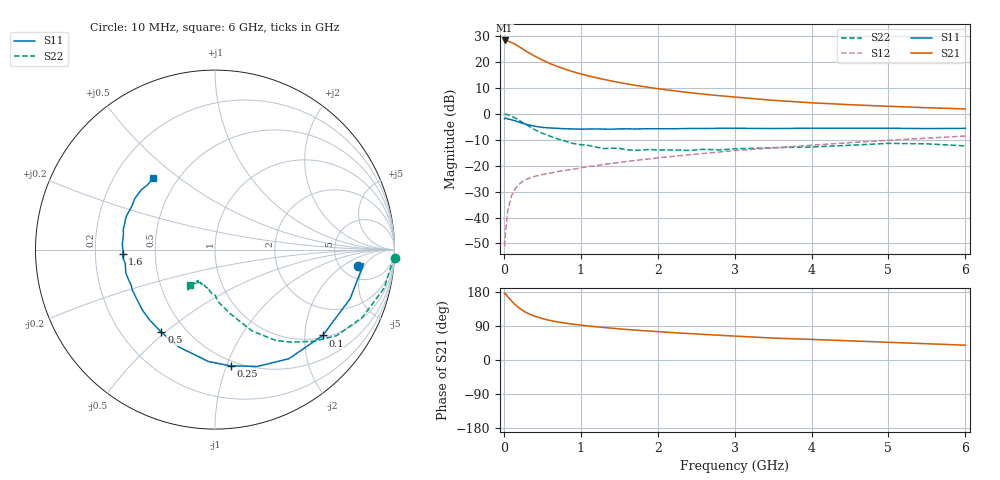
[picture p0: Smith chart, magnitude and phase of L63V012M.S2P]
!  INFINEON TECHNOLOGIES Small Signal Semiconductors
! BFR380L3 , Si-NPN RF-Transistor in TSLP-3-1
!  Vce=3 V,  Ic=12.5 mA
! Common Emitter S-Parameters:  07. March 2005
#  GHz  S  MA  R  50
! f  S11  S21  S12  S22
! GHz  Mag  Ang  Mag  Ang  Mag  Ang  Mag  Ang
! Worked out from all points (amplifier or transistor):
!   36 points, 10 MHz to 6 GHz, reference 50 ohm
!   highest |S21| = 28.4 dB at 10 MHz (marker M1)
!   |S21| within 3 dB of that: start of sweep to 229.8 MHz
!   unconditionally stable (mu >= 1): 2.005 GHz to 4.76 GHz
!   at 250 MHz: K = 0.29, MSG = 25.5 dB, |S12| = -26.0 dB
!   at 1.4 GHz: K = 0.91, MSG = 15.9 dB, |S12| = -19.1 dB
!   at 6 GHz: K = 0.96, MSG = 5.2 dB, |S12| = -8.5 dB
!   S11 on the Smith chart (normalised r, x): 10 MHz: 7.27, -3.66; 100 MHz: 1.06, -2.47; 250 MHz: 0.46, -1.03; 500 MHz: 0.37, -0.49; 1.6 GHz: 0.32, -0.02; 6 GHz: 0.37, +0.40
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0.01  0.8029 -6.4  26.15 175.5  0.0028 85.9  1.004 -2.6
0.02  0.8317 -5.4  26 175.0  0.0049 91.1  0.986 -5.3
0.05  0.8013 -19.9  25.49 167.2  0.0133 81.5  0.9666 -12.8
0.1  0.7678 -38.5  23.86 155.6  0.0264 72.6  0.904 -24.6
0.15  0.7343 -55.9  21.9 145.3  0.0365 65.5  0.8307 -35.2
0.2  0.6923 -70.1  19.72 136.8  0.0439 60.1  0.7505 -42.9
0.25  0.6532 -82.4  17.74 130.2  0.0502 56.3  0.6691 -50.4
0.3  0.6248 -93.3  15.9 124.2  0.0552 53.2  0.6095 -56.2
0.4  0.5787 -110.5  13.07 115.5  0.0622 49.9  0.4981 -65.5
0.5  0.5492 -122.9  10.99 109.4  0.0674 49.0  0.423 -70.9
0.6  0.535 -133.1  9.371 104.4  0.0721 48.8  0.371 -76.2
0.7  0.5261 -140.4  8.204 100.6  0.0771 49.7  0.3292 -80.8
0.9  0.5132 -153.5  6.505 94.5  0.0853 51.2  0.2692 -88.6
1.1  0.5102 -161.5  5.414 89.7  0.0963 53.3  0.2463 -94.0
1.4  0.506 -171.4  4.311 84.1  0.1104 55.5  0.2176 -100.4
1.6  0.5152 -177.3  3.799 80.5  0.1209 56.6  0.2031 -107.9
2.2  0.5168 170.9  2.81 72.2  0.1518 59.5  0.2018 -112.9
2.8  0.5272 161.1  2.247 65.3  0.1839 61.3  0.202 -120.5
3.5  0.5223 152.0  1.828 57.9  0.2207 60.9  0.2229 -121.7
4.5  0.5291 145.0  1.506 50.6  0.2788 61.0  0.2478 -123.3
5.5  0.521 136.3  1.316 42.9  0.3413 58.6  0.2639 -124.4
6  0.5265 130.9  1.247 39.1  0.3745 56.9  0.2414 -126.0
